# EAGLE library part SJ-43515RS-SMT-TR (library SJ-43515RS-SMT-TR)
4 conductor 3.5 mm Surface Mount Audio Jack w/ Ring Switch Source: Datasheet
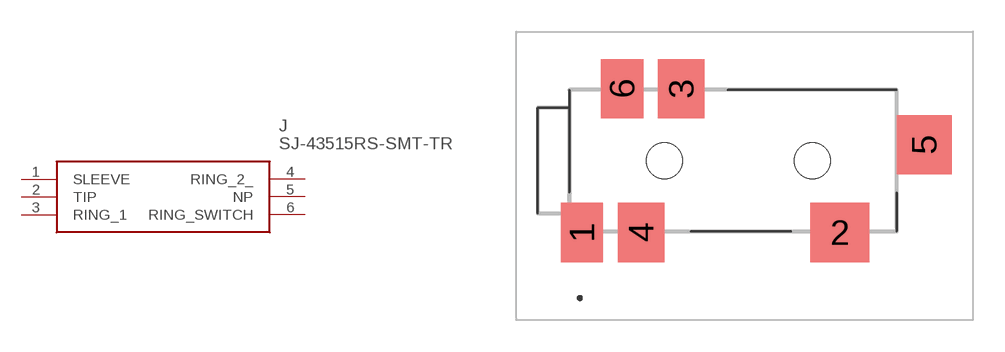
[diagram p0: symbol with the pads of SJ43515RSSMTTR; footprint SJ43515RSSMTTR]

Designator prefix J

## SJ-43515RS-SMT-TR (Arrow_Part_Number: SJ-43515RS-SMT-TR; Arrow_Price-Stock: https://www.arrow.com/en/products/sj-43515rs-smt-tr/cui-devices?region=nac; Description: 4 conductor 3.5 mm Surface Mount Audio Jack w/ Ring Switch; Height: 5.1mm; Manufacturer_Name: CUI Devices; Manufacturer_Part_Number: SJ-43515RS-SMT-TR; Mouser_Part_Number: 490-SJ43515RS-SMT-TR; Mouser_Price-Stock: https://www.mouser.co.uk/ProductDetail/CUI-Devices/SJ-43515RS-SMT-TR?qs=WyjlAZoYn539wol%252BXvq5nw%3D%3D)  [SJ43515RSSMTTR]
1  SLEEVE
2  TIP
3  RING_1
4  RING_2_
5  NP
6  RING_SWITCH

## Footprint SJ43515RSSMTTR (pad centres in mm)
SJ-43515RS-SMT-TR-2
smd 2 x 2.8: 1 -7.7,-3.4; 6 -5.8,3.4
smd 2.8 x 2.8: 2 4.5,-3.4
smd 2.2 x 2.8: 3 -3,3.4; 4 -4.9,-3.4
smd 2.6 x 2.8: 5 8.5,0.75
hole 1.7 at -3.8,0
hole 1.7 at 3.2,0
